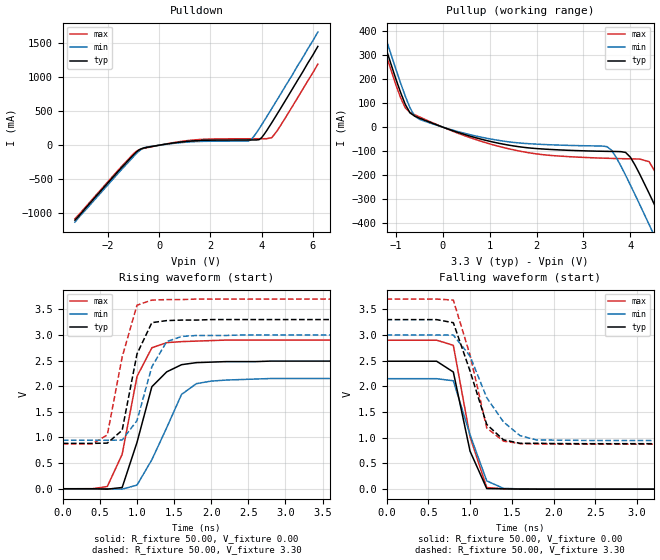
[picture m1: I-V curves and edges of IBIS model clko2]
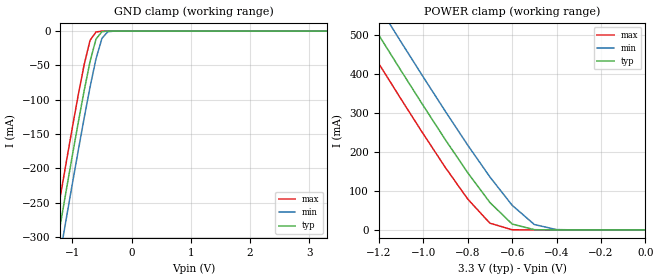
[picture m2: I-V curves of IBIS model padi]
|   * 9112_17.ibs * IBIS 2.1 Model for ICS9112-17
| Rev History
| Rev No.   Description
| 1.0   Initial release with Updated Parasitic Parameters
[IBIS Ver]   2.1
[Comment char]  |_char
[File name]   9112_17.ibs
[Date]   September 05, 2001
[File Rev]   1.1
[Source]   Originated at Integrated Circuit Systems, Inc.
[Disclaimer]
(C) Copyright Integrated Circuit Systems, Inc. 1997
   All rights reserved
ICS hereby grants the user of this IBIS model a non-exclusive,
nontransferable license to use this IBIS model under the following terms.
Before using this IBIS model, the user should read this license.
If the user does not accept these terms,  the IBIS model should be
returned to ICS within 30 days.
   The user is granted this license only to use the IBIS model and
is not granted rights to sell, load, rent, lease or license the IBIS
model in whole or in part, or in modified form to anyone other than
user. User may modify the IBIS model to suit its specific
applications but rights to derivative works and such modifications
shall belong to ICS.
   This IBIS model is provided on an "AS IS" basis and ICS makes
absolutely no warranty with respect to the information contained
herein. ICS DISCLAIMS AND CUSTOMER WAIVES ALL WARRANTIES, EXPRESS
OR IMPLIED, INCLUDING WARRANTIES OF MERCHANTABILITY OR FITNESS FOR
A PARTICULAR PURPOSE. The entire risk as to quality and performance
is with the Customer. ACCORDINGLY, IN NO EVENT SHALL THE COMPANY BE
LIABLE FOR ANY DAMAGES, WHETHER IN CONTRACT OR TORT,INCLUDING ANY
LOST PROFITS OR OTHER INCIDENTAL, CONSEQUENTIAL, EXEMPLARY, OR
PUNITIVE DAMAGES ARISING OUT OF THE USE OR APPLICATION OF THE IBIS
model provided in this package. Further, ICS reserves the right to
make changes without notice to any product herein to improve
reliability, function, or design. ICS does not convey any license
under patent rights or any other intellectual property rights,
including those of third parties.
   ICS is not obligated to provide maintenance or support
for the licensed IBIS model.
|   COMPONENT: ICS9112-17
[Component]   9112-17
[Manufacturer]  ICS
[Package]
| variable   typ   min   max
R_pkg   37.6m   32.9m   42.3m
L_pkg   3.1nH   2.6nH   3.6nH
C_pkg   0.34pF  0.14pF  0.54pF
[Pin]   signal_name   model_name   R_pin   L_pin   C_pin
1   REF   padi
2   CLKA1   clko2
3   CLKA2   clko2
4   VDD   POWER
5   GND   GND
6   CLKB1   clko2
7   CLKB2   clko2
8   FS2   padi
9   FS1   padi
10   CLKB3   clko2
11   CLKB4   clko2
12   GND   GND
13   VDD   POWER
14   CLKA3   clko2
15   CLKA4   clko2
16   CLKOUT   clko2
| Models and submodels in the file (2): clko2 (Output), padi (Input)
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|   Model clko2
[Model]   clko2
Model_type   Output
Polarity   Inverting
Vmeas =   1.40V
Cref =  30.00pF
Rref =  0.000
Vref =   1.40V
C_comp   5.50pF   5.00pF   6.00pF
[Temperature Range]   27.00   70.00   0.00
[Voltage Range]   3.30V   3.00V   3.70V
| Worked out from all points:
|   slope of the pulldown table from 0 to 0.495 V, typ, clamps not added: 16.8 ohm
|   slope of the pullup table from 0 to 0.495 V, typ, clamps not added: 15.3 ohm
|   rising waveform, R_fixture 50.00, V_fixture 0.00: 20-80 % time 294ps typ, 418ps min, 276ps max; typ from 0 V to 2.49 V
|   rising waveform, R_fixture 50.00, V_fixture 3.30: 20-80 % time 231ps typ, 280ps min, 261ps max; typ from 0.885 V to 3.3 V
|   falling waveform, R_fixture 50.00, V_fixture 0.00: 20-80 % time 229ps typ, 266ps min, 235ps max; typ from 2.49 V to 0 V
|   falling waveform, R_fixture 50.00, V_fixture 3.30: 20-80 % time 289ps typ, 380ps min, 263ps max; typ from 3.3 V to 0.885 V
[Pulldown]
| voltage   I(typ)   I(min)   I(max)
-3.3V     -1.1A      -1.13A     -1.08A
-1V       -137.4mA   -163.8mA   -122.4mA
-800mV    -70.43mA   -89.32mA   -68.58mA
-600mV    -40.54mA   -38.22mA   -45.57mA
1.3V      62.76mA    50.25mA    75.08mA
3.4V      76.46mA    60.27mA    94.32mA
3.6V      76.73mA    85.46mA    94.61mA
3.9V      81.28mA    239.3mA    95.03mA
4V        110.4mA    297.6mA    95.17mA
4.4V      331.4mA    538.9mA    110.3mA
4.8V      574.9mA    785.5mA    323.4mA
6.2V      1.45A      1.66A      1.19A
[Pullup]
| voltage   I(typ)   I(min)   I(max)
-3.3V     1.62A      1.66A      1.59A
-1.5V     498.6mA    540.4mA    472.7mA
-1V       199.7mA    240.4mA    175.5mA
-800mV    94.43mA    128.9mA    80.1mA
-500mV    37.58mA    32.76mA    42.73mA
1.5V      -77.83mA   -63.26mA   -94.08mA
3.5V      -100.7mA   -80.93mA   -129.4mA
3.9V      -105.2mA   -200.3mA   -131.4mA
4.4V      -274.8mA   -404.4mA   -143.5mA
4.8V      -440.8mA   -572.5mA   -288.1mA
5.2V      -609.8mA   -742.1mA   -454.3mA
6.2V      -1.04A     -1.17A     -879.8mA
[Ramp]
| variable   typ   min   max
dV/dt_r   1.49/271.03p   1.29/349.40p   1.74/218.41p
dV/dt_f   1.45/200.00p   1.23/300.00p   1.69/200.00p
[Rising Waveform]
R_fixture = 50.00
V_fixture = 0.00
V_fixture_min = 0.00
V_fixture_max = 0.00
| time   V(typ)   V(min)   V(max)
0s        0V         0V         0V
600ps     -8.22mV    294uV      43.46mV
800ps     24.25mV    -7.88mV    671.9mV
1ns       904.8mV    71.09mV    2.19V
1.2ns     1.99V      565.8mV    2.75V
1.4ns     2.28V      1.19V      2.85V
1.6ns     2.42V      1.84V      2.87V
1.8ns     2.46V      2.05V      2.88V
2ns       2.47V      2.1V       2.89V
10ns      2.49V      2.15V      2.9V
[Rising Waveform]
R_fixture = 50.00
V_fixture = 3.30
V_fixture_min = 3.00
V_fixture_max = 3.70
| time   V(typ)   V(min)   V(max)
0s        885.1mV    946.6mV    875.9mV
400ps     885.1mV    946.6mV    876mV
600ps     889.8mV    945.2mV    1.05V
800ps     1.14V      950.5mV    2.57V
1ns       2.63V      1.33V      3.58V
1.2ns     3.24V      2.38V      3.68V
1.4ns     3.28V      2.87V      3.69V
1.6ns     3.29V      2.97V      3.69V
1.8ns     3.29V      2.99V      3.7V
10ns      3.3V       3V         3.7V
[Falling Waveform]
R_fixture = 50.00
V_fixture = 0.00
V_fixture_min = 0.00
V_fixture_max = 0.00
| time   V(typ)   V(min)   V(max)
0s        2.49V      2.15V      2.9V
600ps     2.49V      2.15V      2.9V
800ps     2.28V      2.11V      2.8V
1ns       740.4mV    1.06V      1.02V
1.2ns     10.89mV    161.2mV    31.21mV
1.4ns     6.62mV     16.01mV    7.88mV
1.6ns     2.06mV     4.23mV     1.77mV
10ns      0V         0V         0V
[Falling Waveform]
R_fixture = 50.00
V_fixture = 3.30
V_fixture_min = 3.00
V_fixture_max = 3.70
| time   V(typ)   V(min)   V(max)
0s        3.3V       3V         3.7V
600ps     3.3V       3V         3.7V
800ps     3.24V      3V         3.68V
1ns       2.3V       2.59V      2.61V
1.2ns     1.26V      1.78V      1.19V
1.4ns     960.6mV    1.31V      934.7mV
1.6ns     891.9mV    1.04V      887.1mV
1.8ns     893.2mV    956.5mV    879.9mV
2.8ns     885.2mV    946.2mV    875.9mV
10ns      885.1mV    946.6mV    875.9mV
|   MODEL padi
[Model]   padi
Model_type   Input
Vinl = 800.00mV
Vinh =   2.00V
C_comp   5.5pF   5.0pF   6.0pF
[Voltage range]   3.300   3.000   3.700
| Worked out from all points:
|   GND clamp passes 1 mA (typ) near -0.50 V on its own axis
|   POWER clamp passes 1 mA (typ) near -0.50 V on its own axis
[GND_clamp]
|  Voltage   I(typ)   I(min)   I(max)
-3.3V     -1.37A     -1.409A    -1.331A
-1.3V     -331.8mA   -373.2mA   -290.8mA
-1.2V     -281.3mA   -322.7mA   -240.2mA
-1.1V     -231.2mA   -272.6mA   -190.2mA
-900mV    -133.5mA   -174.4mA   -93.39mA
-800mV    -86.94mA   -126.8mA   -48.84mA
-700mV    -44.15mA   -81.44mA   -13.49mA
-600mV    -11.56mA   -40.46mA   -1.257mA
-500mV    -795uA     -10.56mA   -77.54uA
-400mV    -27.71uA   -852.7uA   -1.223uA
3.3V      227.9pA    44.02uA    159.3pA
[POWER_clamp]
|  Voltage   I(typ)   I(min)   I(max)
-3.3V     2.484A     2.554A     2.415A
-1.3V     592.5mA    666.2mA    519.5mA
-1.2V     500.5mA    574.3mA    427.4mA
-1.1V     409.4mA    483.1mA    336.3mA
-900mV    231.5mA    304.4mA    160.2mA
-800mV    147.3mA    218.1mA    79.55mA
-700mV    70.56mA    136.3mA    17.43mA
-600mV    15.25mA    63.53mA    531.6uA
-500mV    728.2uA    14mA       8.075uA
-400mV    20.89uA    955uA      118.3nA
0V        227.9pA    10.63nA    207.3pA
